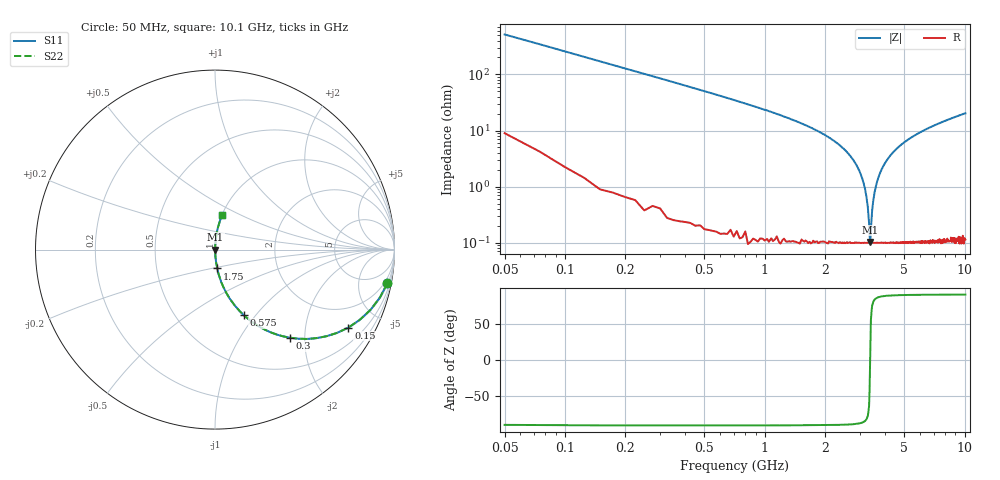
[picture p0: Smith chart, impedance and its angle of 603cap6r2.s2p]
! AVX Thin Film Operation		Date: November 2004
! Description: Accu-P® Series, Thin Film, SMD, RF Capacitor
! Part Number: 06035J6R2BBT
! 50 MHz  -  10.05 GHz
! Serial Measurements
# hz S db R 50
!	S11		S21		S12		S22
!	dB	Phase	dB	Phase	dB	Phase	dB	Phase
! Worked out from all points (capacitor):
!   400 points, 50 MHz to 10.1 GHz, reference 50 ohm
!   read as one part in series: C = 6.2 pF near 100 MHz
!   lowest |Z| = 104 mohm at 3.38 GHz (marker M1)
!   series resonance near 3.373 GHz, so ESL is about 360 pH
!   S11 on the Smith chart (normalised r, x): 50 MHz: 1, -10; 150 MHz: 1.02, -3.41; 300 MHz: 1.01, -1.70; 575 MHz: 1.00, -0.87; 1.75 GHz: 1.00, -0.21; 10.1 GHz: 1.00, +0.40
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5e7  -0.19 -11.0  -14.40 78.0  -14.40 78.0  -0.19 -11.0
1.5e8  -1.30 -30.3  -5.95 59.4  -5.95 59.4  -1.30 -30.3
3e8  -3.80 -49.5  -2.37 40.2  -2.37 40.2  -3.80 -49.5
5.75e8  -8.02 -66.4  -0.76 23.4  -0.76 23.4  -8.02 -66.4
1.73e9  -19.20 -83.2  -0.06 6.3  -0.06 6.3  -19.20 -83.2
1.75e9  -19.50 -83.3  -0.06 6.1  -0.06 6.1  -19.50 -83.3
2.53e9  -27.00 -86.2  -0.02 2.5  -0.02 2.5  -27.00 -86.2
2.98e9  -34.40 -85.9  -0.01 1.1  -0.01 1.1  -34.40 -85.9
3.23e9  -43.50 -81.1  -0.01 0.4  -0.01 0.4  -43.50 -81.1
3.28e9  -47.10 -76.7  -0.01 0.2  -0.01 0.2  -47.10 -76.7
3.33e9  -53.00 -63.2  -0.01 0.1  -0.01 0.1  -53.00 -63.2
3.35e9  -57.60 -40.4  -0.01 0.0  -0.01 0.0  -57.60 -40.4
3.38e9  -59.70 15.7  -0.01 -0.0  -0.01 -0.0  -59.70 15.7
3.4e9  -55.30 54.5  -0.01 -0.1  -0.01 -0.1  -55.30 54.5
3.45e9  -48.50 74.4  -0.01 -0.2  -0.01 -0.2  -48.50 74.4
3.55e9  -41.90 82.4  -0.01 -0.5  -0.01 -0.5  -41.90 82.4
3.8e9  -34.70 85.8  -0.01 -1.1  -0.01 -1.1  -34.70 85.8
4.25e9  -28.90 86.3  -0.01 -2.0  -0.01 -2.0  -28.90 86.3
5.08e9  -23.90 85.4  -0.03 -3.7  -0.03 -3.7  -23.90 85.4
6.75e9  -18.90 82.9  -0.07 -6.5  -0.07 -6.5  -18.90 82.9
8.43e9  -16.00 80.5  -0.12 -9.1  -0.12 -9.1  -16.00 80.5
1.01e10  -14.10 78.3  -0.18 -11.4  -0.18 -11.4  -14.10 78.3
